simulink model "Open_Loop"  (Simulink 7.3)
settings: Solver=ode45  StartTime=0.0  StopTime=2  RelTol=1e-3
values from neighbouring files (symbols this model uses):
  Afc = [    [fcs.m]
  Ave = [    [vehicle.m]    (also in vehicle_eo.m)
  Bfc = [    [fcs.m]
  Bve = [    [vehicle.m]    (also in vehicle_eo.m)
  Cfc = [    [fcs.m]
  Cve = [    [vehicle.m]    (also in vehicle_eo.m)
  Dfc = [    [fcs.m]
  Dve = [    [vehicle.m]    (also in vehicle_eo.m)
  thc = 8    [run.m]
undefined symbols (not defined in the file or in its folder): Aac, Bac, Cac, Dac, ThVC_eo

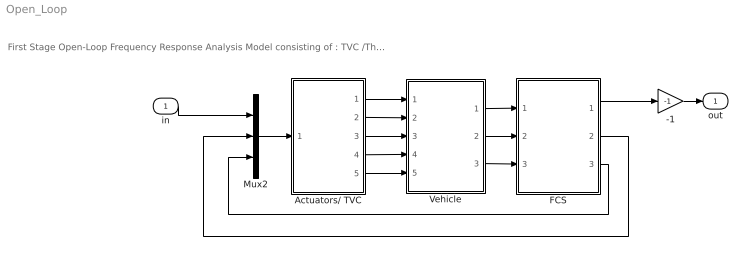
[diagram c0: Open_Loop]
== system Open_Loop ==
  note: First Stage Open-Loop Frequency Response Analysis Model consisting of : TVC /Throttle Control, Actuators, Vehicle, and Flight Control
  in : Inport  OutDataType=sfix(16)  OutScaling=2^0
  -1 : Gain  Gain=-1  ParameterDataType=sfix(16)  ParameterScaling=2^0  OutDataType=sfix(16)  OutScaling=2^0
  Actuators/ TVC : Subsystem
  FCS : Subsystem
  Mux2 : Mux  Inputs=3
  Vehicle : Subsystem
  out : Outport  OutDataType=sfix(16)  OutScaling=2^0
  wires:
  Mux2/1 -> Actuators/ TVC/1(TVC)
  Vehicle/1(atti) -> FCS/1(atti)
  Vehicle/2(rate) -> FCS/2(rate)
  Vehicle/3(accel) -> FCS/3(accel)
  Actuators/ TVC/1(dy (pitch)) -> Vehicle/1(dy)
  Actuators/ TVC/2(dy-ddot) -> Vehicle/2(dy-dd)
  Actuators/ TVC/3(dz (yaw)) -> Vehicle/3(dz)
  Actuators/ TVC/4(dz-ddot) -> Vehicle/4(dz-dd)
  Actuators/ TVC/5(DThrottle) -> Vehicle/5(Dthro)
  -1/1 -> out/1
  FCS/3(Dr_Tvc) -> Mux2/3
  FCS/2(Dq_Tvc) -> Mux2/2
  in/1 -> Mux2/1
  FCS/1(Dp_Tvc) -> -1/1

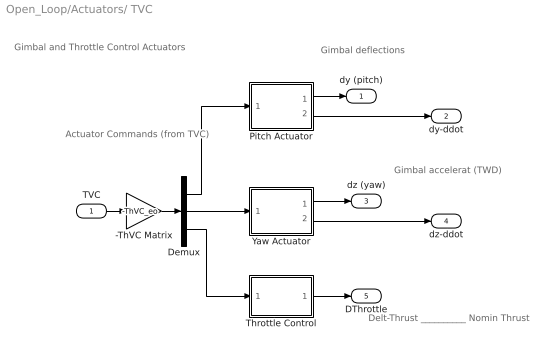
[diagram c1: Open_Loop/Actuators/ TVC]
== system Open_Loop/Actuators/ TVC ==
  note: Delt-Thrust __________ Nomin Thrust
  note: Gimbal accelerat (TWD)
  note: Gimbal deflections
  note: Actuator Commands (from TVC)
  note: Gimbal and Throttle Control Actuators
  TVC : Inport  OutDataType=sfix(16)  OutScaling=2^0
  -ThVC Matrix : Gain  Gain=-ThVC_eo  Multiplication=Matrix(K*u) (u vector)  ParameterDataType=sfix(16)  ParameterScaling=2^0  OutDataType=sfix(16)  OutScaling=2^0
  Demux : Demux  Outputs=[9, 9, 6]
  Pitch Actuator : Subsystem
  Throttle Control : Subsystem
  Yaw Actuator : Subsystem
  dy (pitch) : Outport  OutDataType=sfix(16)  OutScaling=2^0
  dy-ddot : Outport  Port=2  OutDataType=sfix(16)  OutScaling=2^0
  dz (yaw) : Outport  Port=3  OutDataType=sfix(16)  OutScaling=2^0
  dz-ddot : Outport  Port=4  OutDataType=sfix(16)  OutScaling=2^0
  DThrottle : Outport  Port=5  OutDataType=sfix(16)  OutScaling=2^0
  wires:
  Throttle Control/1(tho) -> DThrottle/1
  Yaw Actuator/2(dz-dd) -> dz-ddot/1
  TVC/1 -> -ThVC Matrix/1
  Yaw Actuator/1(dz) -> dz (yaw)/1
  Pitch Actuator/2(dy-dd) -> dy-ddot/1
  Pitch Actuator/1(dy) -> dy (pitch)/1
  Demux/2 -> Yaw Actuator/1(dz-c)
  Demux/1 -> Pitch Actuator/1(dy-c)
  Demux/3 -> Throttle Control/1(thi)
  -ThVC Matrix/1 -> Demux/1

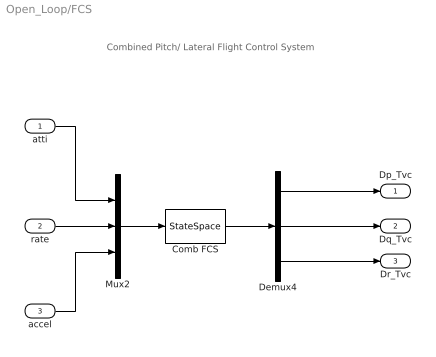
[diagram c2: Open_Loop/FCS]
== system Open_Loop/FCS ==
  note: Combined Pitch/ Lateral Flight Control System
  atti : Inport  OutDataType=sfix(16)  OutScaling=2^0
  rate : Inport  Port=2  OutDataType=sfix(16)  OutScaling=2^0
  accel : Inport  Port=3  OutDataType=sfix(16)  OutScaling=2^0
  Comb FCS : StateSpace  A=Afc  B=Bfc  C=Cfc  D=Dfc
  Demux4 : Demux  Outputs=3
  Mux2 : Mux  Inputs=[3, 3, 2]
  Dp_Tvc : Outport  OutDataType=sfix(16)  OutScaling=2^0
  Dq_Tvc : Outport  Port=2  OutDataType=sfix(16)  OutScaling=2^0
  Dr_Tvc : Outport  Port=3  OutDataType=sfix(16)  OutScaling=2^0
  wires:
  Demux4/3 -> Dr_Tvc/1
  Demux4/1 -> Dp_Tvc/1
  rate/1 -> Mux2/2
  atti/1 -> Mux2/1
  accel/1 -> Mux2/3
  Mux2/1 -> Comb FCS/1
  Comb FCS/1 -> Demux4/1
  Demux4/2 -> Dq_Tvc/1

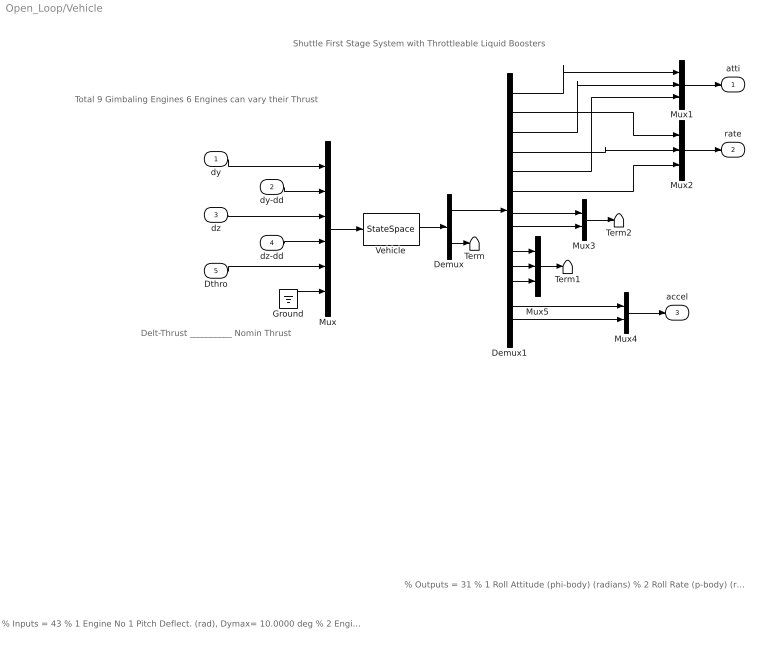
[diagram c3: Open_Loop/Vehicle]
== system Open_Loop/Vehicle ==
  note: Shuttle First Stage System with Throttleable Liquid Boosters
  note: Total 9 Gimbaling Engines 6 Engines can vary their Thrust
  note: Delt-Thrust __________ Nomin Thrust
  note: % Inputs = 43 % 1 Engine No 1 Pitch Deflect. (rad), Dymax= 10.0000 deg % 2 Engine No 2 Pitch Deflect. (rad), Dymax= 10.0000 deg % 3 Engine No 3 Pitch Deflect. (rad), Dymax= 10.0000 deg % 4 Engine No 4 Pitch Deflect. (rad), Dymax= 5.0000 deg % 5 Engine No 5 Pitch Deflect. (rad), Dymax= 5.0000 deg % 6 Engine No 6 Pitch Deflect. (rad), Dymax= 5.0000 deg % 7 Engine No 7 Pitch Deflect. (rad), Dymax= 5.0000 deg % 8 Engine No 8 Pitch Deflect. (rad), Dymax= 5.0000 deg % 9 Engine No 9 Pitch Deflect. (rad), Dymax= 5.0000 deg % 10 Engine No 1 Pitch Acceleration (rad/sec^2) % 11 Engine No 2 Pitch Acceleration (rad/sec^2) % 12 Engine No 3 Pitch Acceleration (rad/sec^2) % 13 Engine No 4 Pitch Acceleration (rad/sec^2) % 14 Engine No 5 Pitch Acceleration (rad/sec^2) % 15 Engine No 6 Pitch Acceleration (rad/sec^2) % 16 Engine No 7 Pitch Acceleration (rad/sec^2) % 17 Engine No 8 Pitch Acceleration (rad/sec^2) % 18 Engine No 9 Pitch Acceleration (rad/sec^2) % 19 Engine No 1 Yaw Deflect. (rad), Dzmax= 10.0000 deg % 20 Engine No 2 Yaw Deflect. (rad), Dzmax= 10.0000 deg % 21 Engine No 3 Yaw Deflect. (rad), Dzmax= 10.0000 deg % 22 Engine No 4 Yaw Deflect. (rad), Dzmax= 1.0000 deg % 23 Engine No 5 Yaw Deflect. (rad), Dzmax= 1.0000 deg % 24 Engine No 6 Yaw Deflect. (rad), Dzmax= 1.0000 deg % 25 Engine No 7 Yaw Deflect. (rad), Dzmax= 1.0000 deg % 26 Engine No 8 Yaw Deflect. (rad), Dzmax= 1.0000 deg % 27 Engine No 9 Yaw Deflect. (rad), Dzmax= 1.0000 deg % 28 Engine No 1 Yaw Acceleration (rad/sec^2) % 29 Engine No 2 Yaw Acceleration (rad/sec^2) % 30 Engine No 3 Yaw Acceleration (rad/sec^2) % 31 Engine No 4 Yaw Acceleration (rad/sec^2) % 32 Engine No 5 Yaw Acceleration (rad/sec^2) % 33 Engine No 6 Yaw Acceleration (rad/sec^2) % 34 Engine No 7 Yaw Acceleration (rad/sec^2) % 35 Engine No 8 Yaw Acceleration (rad/sec^2) % 36 Engine No 9 Yaw Acceleration (rad/sec^2) % 37 Throttle Input dTh/Th for Engine No 4 (-) % 38 Throttle Input dTh/Th for Engine No 5 (-) % 39 Throttle Input dTh/Th for Engine No 
  note: % Outputs = 31 % 1 Roll Attitude (phi-body) (radians) % 2 Roll Rate (p-body) (rad/sec) % 3 Pitch Attitude (thet-bdy) (radians) % 4 Pitch Rate (q-body) (rad/sec) % 5 Yaw Attitude (psi-body) (radians) % 6 Yaw Rate (r-body) (rad/sec) % 7 Angle of attack, alfa, (radians) % 8 Angle of sideslip, beta, (radian) % 9 Change in Altitude, delta-h, (feet) % 10 Forward Acceleration (V-dot) (ft/sec) % 11 Cross Range Velocity (Vcr) (ft/sec) % 12 Accelerom # 1, (along Z), (ft/sec^2) Translat. Acceler % 13 Accelerom # 2, (along Y), (ft/sec^2) Translat. Acceler % 14 Ptch Load-Torque Tly for Engine: 1,(ft-lb) % 15 Ptch Load-Torque Tly for Engine: 2,(ft-lb) % 16 Ptch Load-Torque Tly for Engine: 3,(ft-lb) % 17 Ptch Load-Torque Tly for Engine: 4,(ft-lb) % 18 Ptch Load-Torque Tly for Engine: 5,(ft-lb) % 19 Ptch Load-Torque Tly for Engine: 6,(ft-lb) % 20 Ptch Load-Torque Tly for Engine: 7,(ft-lb) % 21 Ptch Load-Torque Tly for Engine: 8,(ft-lb) % 22 Ptch Load-Torque Tly for Engine: 9,(ft-lb) % 23 Yaw Load-Torque Tlz for Engine: 1,(ft-lb) % 24 Yaw Load-Torque Tlz for Engine: 2,(ft-lb) % 25 Yaw Load-Torque Tlz for Engine: 3,(ft-lb) % 26 Yaw Load-Torque Tlz for Engine: 4,(ft-lb) % 27 Yaw Load-Torque Tlz for Engine: 5,(ft-lb) % 28 Yaw Load-Torque Tlz for Engine: 6,(ft-lb) % 29 Yaw Load-Torque Tlz for Engine: 7,(ft-lb) % 30 Yaw Load-Torque Tlz for Engine: 8,(ft-lb) % 31 Yaw Load-Torque Tlz for Engine: 9,(ft-lb)
  dy : Inport  OutDataType=sfix(16)  OutScaling=2^0
  dy-dd : Inport  Port=2  OutDataType=sfix(16)  OutScaling=2^0
  dz : Inport  Port=3  OutDataType=sfix(16)  OutScaling=2^0
  dz-dd : Inport  Port=4  OutDataType=sfix(16)  OutScaling=2^0
  Dthro : Inport  Port=5  OutDataType=sfix(16)  OutScaling=2^0
  Demux : Demux  Outputs=[13,18]
  Demux1 : Demux  Outputs=13
  Ground : Ground
  Mux : Mux  Inputs=[9, 9, 9, 9, 6, 1]
  Mux1 : Mux  Inputs=3
  Mux2 : Mux  Inputs=3
  Mux3 : Mux  Inputs=2
  Mux4 : Mux  Inputs=2
  Mux5 : Mux  Inputs=3
  Term : Terminator
  Term1 : Terminator
  Term2 : Terminator
  Vehicle : StateSpace  A=Ave  B=Bve  C=Cve  D=Dve
  atti : Outport  OutDataType=sfix(16)  OutScaling=2^0
  rate : Outport  Port=2  OutDataType=sfix(16)  OutScaling=2^0
  accel : Outport  Port=3  OutDataType=sfix(16)  OutScaling=2^0
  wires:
  Mux1/1 -> atti/1
  Mux5/1 -> Term1/1
  Demux1/11 -> Mux5/3
  Demux1/10 -> Mux5/2
  Demux1/9 -> Mux5/1
  Dthro/1 -> Mux/5
  dz-dd/1 -> Mux/4
  dz/1 -> Mux/3
  dy-dd/1 -> Mux/2
  dy/1 -> Mux/1
  Mux4/1 -> accel/1
  Mux2/1 -> rate/1
  Demux1/13 -> Mux4/2
  Demux1/12 -> Mux4/1
  Demux1/8 -> Mux3/2
  Demux1/7 -> Mux3/1
  Demux1/6 -> Mux2/3
  Demux1/4 -> Mux2/2
  Demux1/2 -> Mux2/1
  Demux1/5 -> Mux1/3
  Demux1/3 -> Mux1/2
  Demux1/1 -> Mux1/1
  Demux/2 -> Term/1
  Demux/1 -> Demux1/1
  Vehicle/1 -> Demux/1
  Mux/1 -> Vehicle/1
  Mux3/1 -> Term2/1
  Ground/1 -> Mux/6

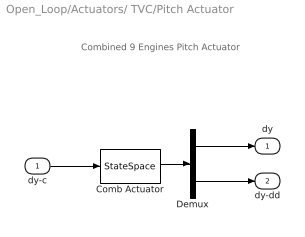
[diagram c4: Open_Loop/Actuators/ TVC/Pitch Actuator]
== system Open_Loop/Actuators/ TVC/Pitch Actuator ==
  note: Combined 9 Engines Pitch Actuator
  dy-c : Inport  OutDataType=sfix(16)  OutScaling=2^0
  Comb Actuator : StateSpace  A=Aac  B=Bac  C=Cac  D=Dac
  Demux : Demux  Outputs=[9, 9]
  dy : Outport  OutDataType=sfix(16)  OutScaling=2^0
  dy-dd : Outport  Port=2  OutDataType=sfix(16)  OutScaling=2^0
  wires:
  dy-c/1 -> Comb Actuator/1
  Demux/2 -> dy-dd/1
  Demux/1 -> dy/1
  Comb Actuator/1 -> Demux/1

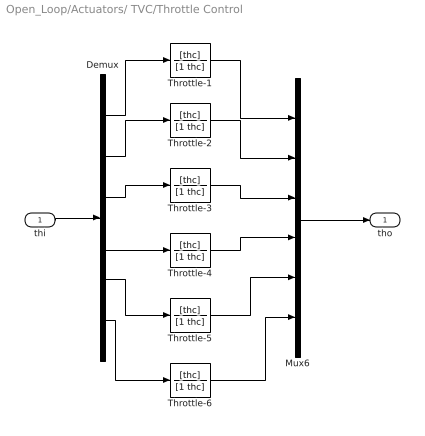
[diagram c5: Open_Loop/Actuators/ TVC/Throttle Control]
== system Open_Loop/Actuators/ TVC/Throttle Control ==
  thi : Inport  OutDataType=sfix(16)  OutScaling=2^0
  Demux : Demux  Outputs=6
  Mux6 : Mux  Inputs=6
  Throttle-{1..6} (6 alike) : TransferFcn  Numerator=[thc]  Denominator=[1 thc]
  tho : Outport  OutDataType=sfix(16)  OutScaling=2^0
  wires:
  Throttle-6/1 -> Mux6/6
  Throttle-5/1 -> Mux6/5
  Throttle-4/1 -> Mux6/4
  Throttle-3/1 -> Mux6/3
  Throttle-2/1 -> Mux6/2
  Throttle-1/1 -> Mux6/1
  Mux6/1 -> tho/1
  thi/1 -> Demux/1
  Demux/6 -> Throttle-6/1
  Demux/5 -> Throttle-5/1
  Demux/4 -> Throttle-4/1
  Demux/3 -> Throttle-3/1
  Demux/2 -> Throttle-2/1
  Demux/1 -> Throttle-1/1

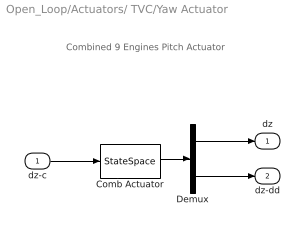
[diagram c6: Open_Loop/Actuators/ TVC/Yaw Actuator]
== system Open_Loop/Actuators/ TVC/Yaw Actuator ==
  note: Combined 9 Engines Pitch Actuator
  dz-c : Inport  OutDataType=sfix(16)  OutScaling=2^0
  Comb Actuator : StateSpace  A=Aac  B=Bac  C=Cac  D=Dac
  Demux : Demux  Outputs=[9, 9]
  dz : Outport  OutDataType=sfix(16)  OutScaling=2^0
  dz-dd : Outport  Port=2  OutDataType=sfix(16)  OutScaling=2^0
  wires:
  dz-c/1 -> Comb Actuator/1
  Demux/2 -> dz-dd/1
  Demux/1 -> dz/1
  Comb Actuator/1 -> Demux/1
